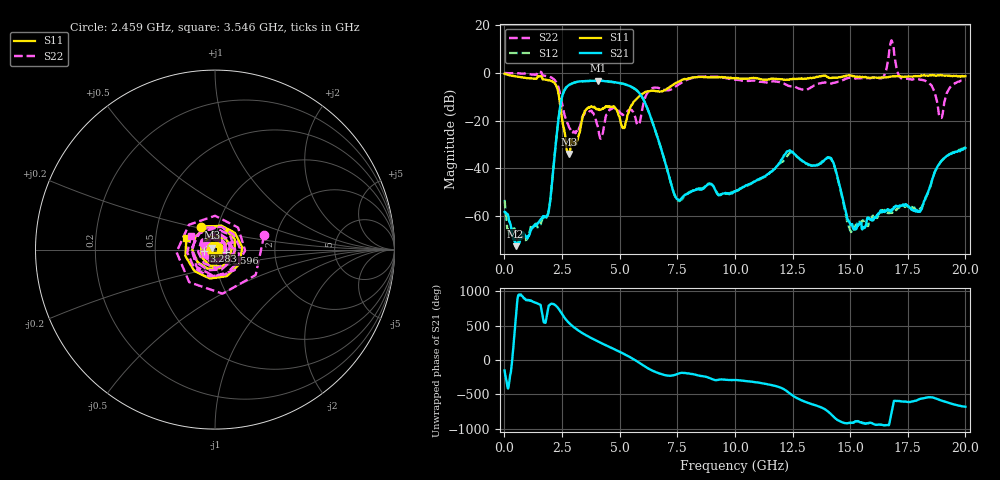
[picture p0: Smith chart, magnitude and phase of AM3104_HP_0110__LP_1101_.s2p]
!Created with skrf (http://scikit-rf.org).
# Hz S RI R 50.0
!freq ReS11 ImS11 ReS21 ImS21 ReS12 ImS12 ReS22 ImS22
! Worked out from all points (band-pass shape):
!   1601 points, 10 MHz to 20 GHz, reference 50 ohm
!   highest |S21| = -3.22 dB at 4.083 GHz (marker M1); lowest = -72.5 dB at 484.8 MHz (marker M2)
!   |S21| within 3 dB of the highest: 2.672 GHz to 5.59 GHz (2.917 GHz wide, 70.6 % of centre)
!   lowest |S11| = -33.9 dB at 2.809 GHz (marker M3), VSWR 1.04, Z = 48.3 + j1.08 ohm
!   |S11| at or under -10 dB: 2.372 GHz to 5.818 GHz (3.446 GHz wide, 84.2 % of centre)
!   |S22| runs from -27.5 to 13.6 dB; largest |S21 - S12| = 0.07
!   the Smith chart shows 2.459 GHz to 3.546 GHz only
!   S11 on the Smith chart (normalised r, x): 2.459 GHz: 0.83, +0.22; 2.596 GHz: 1.13, -0.04; 3.283 GHz: 0.88, -0.01; 3.546 GHz: 0.72, +0.09
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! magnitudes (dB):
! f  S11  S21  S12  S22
! 10 MHz  -0.3  -58.2  -53.1  0.0
! 484.8 MHz  -1.4  -72.5  -67.7  -0.1
! 1.872 GHz  -3.0  -59.6  -59.5  -1.4
! 2.459 GHz  -16.5  -12.0  -12.0  -10.9
! 2.596 GHz  -24.0  -7.4  -7.4  -17.1
! 2.809 GHz  -33.9  -5.0  -5.1  -22.8
! 3.283 GHz  -24.1  -3.5  -3.6  -22.1
! 3.346 GHz  -20.7  -3.5  -3.6  -19.9
! 3.546 GHz  -15.3  -3.4  -3.4  -16.2
! 4.083 GHz  -15.1  -3.2  -3.3  -24.1
! 5.157 GHz  -22.9  -4.5  -4.5  -17.5
! 5.782 GHz  -10.4  -7.6  -7.7  -21.8
! 6.682 GHz  -7.7  -28.1  -28.1  -6.3
! 7.519 GHz  -3.8  -52.9  -53.4  -5.1
! 10.01 GHz  -2.3  -49.8  -49.6  -2.9
! 13.34 GHz  -2.2  -38.8  -38.9  -5.8
! 14.22 GHz  -2.1  -36.6  -36.8  -4.3
! 15.04 GHz  -1.1  -63.6  -66.4  -2.0
! 16.68 GHz  -1.6  -57.5  -58.8  7.3
! 18.03 GHz  -1.4  -57.8  -56.9  -2.8
! 18.93 GHz  -0.8  -37.3  -37.3  -18.8
! 20 GHz  -1.4  -31.5  -31.3  -2.8
